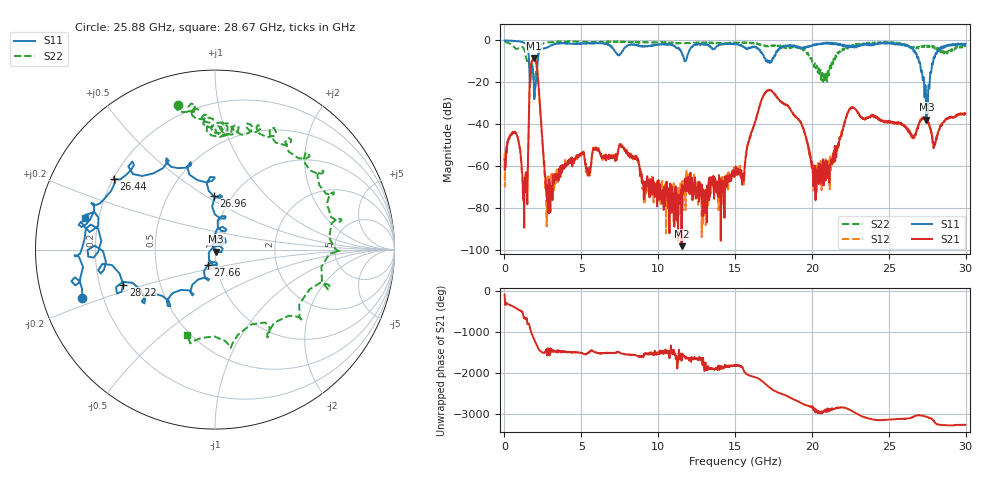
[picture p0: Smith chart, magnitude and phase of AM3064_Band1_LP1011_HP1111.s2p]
# Hz S DB R 50.0
!freq dBS11 angS11 dBS21 angS21 dBS12 angS12 dBS22 angS22
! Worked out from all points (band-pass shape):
!   1600 points, 10 MHz to 29.98 GHz, reference 50 ohm
!   highest |S21| = -8.62 dB at 1.922 GHz (marker M1); lowest = -98.4 dB at 11.52 GHz (marker M2)
!   |S21| within 3 dB of the highest: 1.732 GHz to 2.09 GHz (357.4 MHz wide, 18.7 % of centre)
!   lowest |S11| = -37.9 dB at 27.45 GHz (marker M3), VSWR 1.03, Z = 50.7 - j1.08 ohm
!   |S11| at or under -10 dB: 1.6 GHz to 2.165 GHz (565.1 MHz wide, 30 % of centre); 17.22 GHz to 17.32 GHz (100.8 MHz wide, 0.583 % of centre); 26.95 GHz to 27.89 GHz (939.6 MHz wide, 3.43 % of centre)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
!   |S22| runs from -26.7 to -0.3 dB; largest |S21 - S12| = 0.0064
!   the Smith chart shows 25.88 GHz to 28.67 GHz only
!   S11 on the Smith chart (normalised r, x): 25.88 GHz: 0.12, -0.17; 26.44 GHz: 0.20, +0.30; 26.96 GHz: 0.83, +0.54; 27.66 GHz: 0.91, -0.16; 28.22 GHz: 0.30, -0.17; 28.67 GHz: 0.15, +0.12
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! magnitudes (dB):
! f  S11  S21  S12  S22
! 10 MHz  -0.1  -56.7  -53.9  -0.3
! 741 MHz  -0.3  -44.5  -44.1  -4.0
! 1.36 GHz  -1.5  -67.3  -67.5  -6.6
! 1.734 GHz  -14.7  -11.5  -11.4  -11.9
! 1.922 GHz  -24.4  -8.6  -8.6  -21.1
! 2.84 GHz  -3.2  -70.9  -68.5  -1.0
! 5.015 GHz  -1.5  -54.9  -54.3  -0.7
! 10 GHz  -2.0  -69.0  -70.5  -1.0
! 11.52 GHz  -5.9  -98.4  -71.7  -1.3
! 15 GHz  -1.8  -62.5  -60.9  -1.3
! 17.22 GHz  -9.8  -23.8  -23.8  -2.5
! 19.99 GHz  -2.7  -60.8  -58.7  -9.2
! 22.56 GHz  -2.7  -32.4  -32.2  -3.2
! 25 GHz  -1.1  -38.9  -38.9  -1.1
! 25.88 GHz  -2.1  -40.2  -39.8  -1.6
! 26.44 GHz  -3.3  -45.3  -45.6  -3.3
! 26.96 GHz  -10.5  -40.1  -39.9  -3.2
! 27.45 GHz  -37.9  -37.4  -37.6  -2.5
! 27.66 GHz  -20.3  -40.8  -40.6  -2.9
! 28.22 GHz  -5.2  -43.5  -44.1  -4.9
! 28.67 GHz  -2.6  -38.1  -38.1  -6.0
! 29.98 GHz  -1.6  -35.0  -35.1  -3.1
